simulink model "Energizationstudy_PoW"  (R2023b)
settings: Solver=ode15s  StartTime=0.0  StopTime=25  RelTol=1e-3
PreLoadFcn:
  | Ts=50e-6;
undefined symbols (not defined in the file or in its folder): DiscIntNeverNeededParam, find_system
libraries: spsThreePhaseVIMeasurementLib x11, spsBreakerLib x6, spsabctodq0Lib x6, slpidlib x4, spsFirstOrderFilterLib x3, spsPower3phInstantaneousLib x3, simulink x3, spsThreePhaseBreakerLib x3, spsThreePhaseSeriesRLCBranchLib x2, simulink_extras x2, spsStairGeneratorLib x2, spsThreePhaseSeriesRLCLoadLib x2
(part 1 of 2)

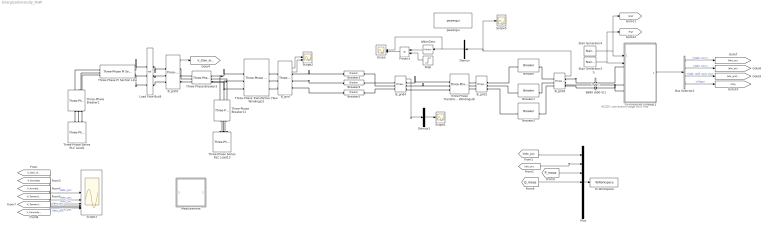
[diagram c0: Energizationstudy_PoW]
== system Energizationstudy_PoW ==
  note: AC/DC conversion stage 80.0 MW
  note: Ts
  B690 (690 V)1 : spsThreePhaseVIMeasurementLib/Three-Phase V-I Measurement  VoltageMeasurement=phase-to-ground  SetLabelV=on  LabelV=Vabc_B575  Vpu=off  VpuLL=off  CurrentMeasurement=yes  SetLabelI=on  LabelI=Iabc_B575  Ipu=off  Pbase=5*2e6/0.9  Vbase=575  OutputType=Complex  PhasorSimulation=off  PSBequivalent=0
  B_grid : spsThreePhaseVIMeasurementLib/Three-Phase V-I Measurement  VoltageMeasurement=phase-to-ground  SetLabelV=off  LabelV=Vabc  Vpu=on  VpuLL=off  CurrentMeasurement=yes  SetLabelI=off  LabelI=Iabc  Ipu=on  Pbase=5e6  Vbase=66e3  OutputType=Complex  PhasorSimulation=off  PSBequivalent=0
  B_grid1 : spsThreePhaseVIMeasurementLib/Three-Phase V-I Measurement  VoltageMeasurement=phase-to-ground  SetLabelV=off  LabelV=Vabc  Vpu=on  VpuLL=off  CurrentMeasurement=yes  SetLabelI=off  LabelI=Iabc  Ipu=on  Pbase=100e6  Vbase=690  OutputType=Complex  PhasorSimulation=off  PSBequivalent=0
  B_grid2 : spsThreePhaseVIMeasurementLib/Three-Phase V-I Measurement  VoltageMeasurement=phase-to-ground  SetLabelV=off  LabelV=Vabc  Vpu=on  VpuLL=off  CurrentMeasurement=no  SetLabelI=off  LabelI=Iabc  Ipu=off  Pbase=5e6  Vbase=132e3  OutputType=Complex  PhasorSimulation=off  PSBequivalent=0
  B_grid3 : spsThreePhaseVIMeasurementLib/Three-Phase V-I Measurement  VoltageMeasurement=phase-to-ground  SetLabelV=off  LabelV=Vabc  Vpu=on  VpuLL=off  CurrentMeasurement=yes  SetLabelI=off  LabelI=Iabc  Ipu=on  Pbase=100e6  Vbase=690  OutputType=Complex  PhasorSimulation=off  PSBequivalent=0
  B_grid4 : spsThreePhaseVIMeasurementLib/Three-Phase V-I Measurement  VoltageMeasurement=phase-to-ground  SetLabelV=off  LabelV=Vabc  Vpu=on  VpuLL=off  CurrentMeasurement=yes  SetLabelI=off  LabelI=Iabc  Ipu=on  Pbase=100e6  Vbase=690  OutputType=Complex  PhasorSimulation=off  PSBequivalent=0
  Breaker : spsBreakerLib/Breaker  InitialState=0  SwitchingTimes=2.0167  External=off  BreakerResistance=0.000001  SnubberResistance=1e6  SnubberCapacitance=1e7  Measurements=None  MoreParameters=on  NoBreakLoop=off
  Breaker1 : spsBreakerLib/Breaker  InitialState=0  SwitchingTimes=2.0117  External=off  BreakerResistance=0.0000001  SnubberResistance=1e6  SnubberCapacitance=1e7  Measurements=None  MoreParameters=on  NoBreakLoop=off
  Breaker2 : spsBreakerLib/Breaker  InitialState=0  SwitchingTimes=2.0117+(0.02/4)  External=off  BreakerResistance=0.0000001  SnubberResistance=1e6  SnubberCapacitance=1e7  Measurements=None  MoreParameters=on  NoBreakLoop=off
  Breaker3 : spsBreakerLib/Breaker  InitialState=0  SwitchingTimes=3.012+0.02/4  External=off  BreakerResistance=0.000001  SnubberResistance=1e6  SnubberCapacitance=1e7  Measurements=None  MoreParameters=on  NoBreakLoop=off
  Breaker4 : spsBreakerLib/Breaker  InitialState=0  SwitchingTimes=3.012  External=off  BreakerResistance=0.000001  SnubberResistance=1e6  SnubberCapacitance=1e7  Measurements=None  MoreParameters=on  NoBreakLoop=off
  Breaker5 : spsBreakerLib/Breaker  InitialState=0  SwitchingTimes=3.012+0.02/4  External=off  BreakerResistance=0.000001  SnubberResistance=1e6  SnubberCapacitance=1e7  Measurements=None  MoreParameters=on  NoBreakLoop=off
  Bus Selector1 : BusSelector  OutputSignals=Vabc_pcc,Iabc_pcc,Iabc_grid_conv_pu,Freq
  Demux : Demux  Outputs=3
  Demux1 : Demux  Outputs=3
  Grid forming inverter1 : Subsystem  LoadFcn=%find_system(gcs,'FollowLinks', 'on', 'LookUnderMasks', 'all');  mask(Grid forming inverter){Vnom=690, fnom=50, Pnom=100e6, Lf=95e-6/20, Rf=10e-3/20, Cf=20*1e-3, Vdc_nom=2000, Innerloops=Inner loops, Kp_cc=0.1425/20, Ki_cc=15/20, Kffv=1, Kp_vc=20*14.25, Ki_vc=20*1500, Kffi=0.9, Virtualimpedance=No virtual impedance, Rvir=0.15, Lvir=50e-5/20, ControlType=Virtual Synchronous Machine, mp=(0.7855e-6)/(2*3.14*50*20), nq=0.5*4.3125e-07/20, Ki_q=1e-4, tau=0.001, Ts=5e-5}
      mask prompts: Vnom "Grid-side converter nominal AC voltage (V):"; fnom "Grid frequency (Hz)"; Pnom "Nominal power (VA)"; Lf "Filter inductance (H)"; Rf "Filter resistance (Ω)"; Cf "Filter capacitor (F):"; Vdc_nom "Nominal DC bus voltage (V)"; Innerloops "Inner loops"; Kp_cc "Proportional gain of the current controller"; Ki_cc "Integral gain of the current controller"; Kffv "Voltage feed-forward"; Kp_vc "Proportional gain of the voltage controller"; Ki_vc "Integral gain of the voltage controller"; Kffi "Current feed-forward"; Virtualimpedance "Virtual impedance"; Rvir "Resistance of the virtual impedance"; Lvir "Inductance of the virtual impedance"; ControlType "Primary control"; mp "P - ω Droop coefficient"; nq "Q - V Droop coefficient"; Ki_q "Integral gain of the reactive power controller"; tau "Filter time constant (s)"; Ts "Sample time (s):"
      mask help: This block implements a model of a grid forming inverter with either droop or virtual synchronous generator control.
      mask init:
      | % Converters data
      | Q_filter=50;
      | 
      | % Controller data
      | Freq_filter=10000;   %Hz
      | Zeta_filter=0.707;
      | Mod_index_max=1.1;
      | T_speed=5;      %Speed reference time constant (s)
      | Iq_ref_limit_time_constant=0.3; %(s)
      | Current_reg_output_limit=1.1;   %(pu)
      | Var_reg_output_hi_limit=1.1;    %(pu)
      | Var_reg_output_low_limit=0.9;   %(pu)
      | Pitch_time_constant=0.01;       %(s)
      | Vf_limit=10;    %Field voltage limit (pu)
      | Freq_sawtooth=2000; %Hz, Boost converter
      | Freq_PWM=3000; %Hz, Inverter
      | Ts_snub=50e-6;  %Sample time to compute snubber resistance
  IsNonZero : simulink/Logic and Bit Operations/Compare To Zero  relop=~=  OutDataTypeStr=boolean
  Load Flow Bus9 : spsLoadFlowBusLib/Load Flow Bus  LConnTagsString=a|b|c  RConnTagsString=a|b|c  Phases=ABC  Connectors=on both sides  ID=Glen Innes 132  Vbase=132e3  Vref=1  Vangle=0  VLF=1  VLFb=1  VLFc=1  angleLF=0  angleLFb=0  angleLFc=0
  Measurement : Subsystem
  Mux : Mux  Inputs=7
  Product : Product
  Scope : Scope  NumInputPorts=2
  Scope1 : Scope
  Scope2 : Scope  NumInputPorts=3
  Scope3 : Scope  NumInputPorts=6
  Scope5 : Scope
  Stair Generator3 : spsStairGeneratorLib/Stair Generator  t=[0]  e=[0]  Ts=0
  Stair Generator4 : spsStairGeneratorLib/Stair Generator  t=[10]  e=[100]  Ts=0
  Step : Step  SampleTime=0
  Three-Phase PI Section Line : spsThreePhasePISectionLineLib/Three-Phase PI Section Line  LConnTagsString=a|b|c  RConnTagsString=A|B|C  Length=1  Frequency=50  Resistances=[14.13/100 44.25/100]  Inductances=[0.0012/100 00.0036/100]  Capacitances=[ 0.0865e-5/100 0.0642e-5/100]
  Three-Phase Series RLC Load1 : spsThreePhaseSeriesRLCLoadLib/Three-Phase Series RLC Load  LConnTagsString=A|B|C  Configuration=Y (grounded)  NominalVoltage=(132000)*1  Vabc=[1e3 1e3 1e3]  Vabcp=[1e3 1e3 1e3]  NominalFrequency=50  UnbalancedPower=off  ActivePower=10e6  InductivePower=0  CapacitivePower=0  Pabc=[10e3 9e3 11e3]  QLabc=[100 90 110]  QCabc=[100 90 110]  Pabcp=[10e3 9e3 11e3]  QLabcp=[100 90 110]  QCabcp=[100 90 110]  Measurements=None  LoadType=constant PQ
  Three-Phase Series RLC Load13 : spsThreePhaseSeriesRLCLoadLib/Three-Phase Series RLC Load  LConnTagsString=A|B|C  Configuration=Y (grounded)  NominalVoltage=(132000)*1  Vabc=[1e3 1e3 1e3]  Vabcp=[1e3 1e3 1e3]  NominalFrequency=50  UnbalancedPower=off  ActivePower=12500  InductivePower=0  CapacitivePower=0  Pabc=[10e3 9e3 11e3]  QLabc=[100 90 110]  QCabc=[100 90 110]  Pabcp=[10e3 9e3 11e3]  QLabcp=[100 90 110]  QCabcp=[100 90 110]  Measurements=None  LoadType=constant PQ
  Three-Phase Transformer (Two Windings)2 : spsThreePhaseTransformerTwoWindingsLib/Three-Phase Transformer (Two Windings)  Winding1Connection=Yg  Winding2Connection=Yg  CoreType=Three-limb core (core-type)  SetSaturation=on  Hysteresis=off  DataFile='hysteresis'  SetInitialFlux=on  Measurements=All measurements (V I Fluxes)  UNITS=pu  NominalPower=[ 100e6 , 50 ]  Winding1=[132e3 , 0.000 , 0.09 ]  Winding2=[ 66e3 , 0.000 , 0.09 ]  Rm=500  Lm=500  L0=0.5  Saturation=[ 0,0 ; 0.0024,1.2 ; 1.0,1.52 ]  InitialFluxes=[-0.7 0 0.7]  BreakLoop=off  DiscreteSolver=Trapezoidal robust  DataType=off  TransfoNumber=1
  Three-Phase Transformer (Two Windings)6 : spsThreePhaseTransformerTwoWindingsLib/Three-Phase Transformer (Two Windings)  Winding1Connection=Yg  Winding2Connection=Yg  CoreType=Three-limb core (core-type)  SetSaturation=on  Hysteresis=off  DataFile='hysteresis'  SetInitialFlux=on  Measurements=All measurements (V I Fluxes)  UNITS=pu  NominalPower=[ 100e6 , 50 ]  Winding1=[66e3 , 0.002 , 0.08 ]  Winding2=[ 690 , 0.002 , 0.08 ]  Rm=500  Lm=500  L0=0.5  Saturation=[ 0,0 ; 0.0024,1.2 ; 1.0,1.52 ]  InitialFluxes=[-0.7 0 0.7]  BreakLoop=off  DiscreteSolver=Trapezoidal robust  DataType=off  TransfoNumber=1
  Three-Phase Breaker1 : spsThreePhaseBreakerLib/Three-Phase Breaker  InitialState=open  SwitchA=on  SwitchB=on  SwitchC=on  SwitchTimes=[120]  External=off  BreakerResistance=1e-10  SnubberResistance=1e10  SnubberCapacitance=inf  Measurements=None
  Three-Phase Breaker11 : spsThreePhaseBreakerLib/Three-Phase Breaker  InitialState=open  SwitchA=on  SwitchB=on  SwitchC=on  SwitchTimes=[120]  External=off  BreakerResistance=1e-10  SnubberResistance=1e10  SnubberCapacitance=inf  Measurements=Breaker currents
  Three-Phase Breaker3 : spsThreePhaseBreakerLib/Three-Phase Breaker  InitialState=open  SwitchA=on  SwitchB=on  SwitchC=on  SwitchTimes=[120]  External=off  BreakerResistance=1e-10  SnubberResistance=1e10  SnubberCapacitance=inf  Measurements=None
  To Workspace : ToWorkspace  VariableName=simout  SaveFormat=Timeseries  SampleTime=-1
  powergui : spspowerguiLib/powergui  SimulationMode=Discrete  SampleTime=5e-5  frequency=50  Iterations=50  frequencyindice=0  Pbase=100e6  ErrMax=1e-4  UnitsV=kV  UnitsW=MW  buscounter=0  FunctionMessages=off  echomessages=off  EnableUseOfTLC=off  CurrentSourceSwitches=off  DisableSnubberDevices=off  DisableRonSwitches=off  DisableVfSwitches=off  DisplayEquations=off  AutomaticDiscreteSolvers=off  SolverType=Tustin  Interpol=off  ExternalGateDelay=off  methode=off  Ts=0  x0status=blocks  SPID=off  SwTol=0  HookPort=off  NonlinearTolerance=1e-4  nMaxIteration=100  ContinueOnMaxIteration=off  RestoreLinks=warning  ResistiveCurrentMeasurement=off  Frange=[0:2:500]  Ylog=off  Xlog=on  ShowGrid=off  save=off  variable=ZData  structure=0  ZoomFFT=on  StartTime=0.0  cycles=1  DisplayStyle=1  fundamental=60  FreqAxis=off  MaxFrequency=1000  frequencyindicesteady=1  RmsSteady=1  display=off
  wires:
  B_grid/1 -> Scope2/1
  B_grid/2 -> Scope2/3
  [Iabc_pcc] -> Mux/2
  Mux/1 -> To Workspace/1
  [Vabc_pcc] -> Mux/1
  B_grid2/1 -> [V_Glen_Innes]
  [V_Glen_Innes] -> Scope3/1  "Vabc_pcc"
  [V_Armidale] -> Scope3/2  "Vabc_pcc"
  [V_Armidale_330] -> Scope3/3  "Vabc_pcc"
  [V_Tamworth_330] -> Scope3/4  "Vabc_pcc"
  [V_Tamworth_132] -> Scope3/5  "Vabc_pcc"
  [V_Gunnedah_132] -> Scope3/6  "Vabc_pcc"
  [Q_meas] -> Mux/4
  [P_meas] -> Mux/3
  Bus Selector1/2 -> [Iabc_pcc]  "<Iabc_pcc>"
  Stair Generator3/1 -> [Pref], Grid forming inverter1/2(Pref_pu)
  Bus Selector1/3 -> [Iabc_grid_conv_pu]  "<Iabc_grid_conv_pu>"
  Grid forming inverter1/1(m) -> Bus Selector1/1
  Bus Selector1/4 -> [Freq]  "<Freq>"
  Bus Selector1/1 -> [Vabc_pcc]  "<Vabc_pcc>"
  Stair Generator4/1 -> [Qref], Grid forming inverter1/1(Qref_pu)
  Demux/2 -> IsNonZero/1, Scope/1
  IsNonZero/1 -> Product/1
  Step/1 -> Product/2
  Product/1 -> Scope/2
  B_grid3/1 -> Scope5/1, Demux/1
  Demux1/2 -> Scope1/1
  B_grid4/1 -> Demux1/1
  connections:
  B_grid/LConn1 -- Three-Phase Transformer (Two Windings)2/RConn1
  B_grid/LConn2 -- Three-Phase Transformer (Two Windings)2/RConn2
  B_grid/LConn3 -- Three-Phase Transformer (Two Windings)2/RConn3
  Three-Phase Breaker3/RConn1 -- Three-Phase Breaker11/LConn1 -- Three-Phase Transformer (Two Windings)2/LConn1
  Three-Phase Breaker11/RConn3 -- Three-Phase Series RLC Load13/LConn1
  Three-Phase Breaker11/RConn2 -- Three-Phase Series RLC Load13/LConn2
  Three-Phase Breaker11/RConn1 -- Three-Phase Series RLC Load13/LConn3
  Three-Phase PI Section Line/LConn2 -- Three-Phase Breaker1/LConn2
  Three-Phase Breaker1/LConn1 -- Three-Phase PI Section Line/LConn1
  Three-Phase Breaker1/LConn3 -- Three-Phase PI Section Line/LConn3
  Three-Phase PI Section Line/RConn1 -- Load Flow Bus9/RConn1
  Three-Phase PI Section Line/RConn2 -- Load Flow Bus9/RConn2
  Three-Phase PI Section Line/RConn3 -- Load Flow Bus9/RConn3
  Three-Phase Transformer (Two Windings)6/RConn1 -- B_grid1/LConn1
  Three-Phase Transformer (Two Windings)6/RConn2 -- B_grid1/LConn2
  Three-Phase Transformer (Two Windings)6/RConn3 -- B_grid1/LConn3
  Load Flow Bus9/LConn1 -- B_grid2/LConn1
  Load Flow Bus9/LConn2 -- B_grid2/LConn2
  Load Flow Bus9/LConn3 -- B_grid2/LConn3
  B_grid2/RConn1 -- Three-Phase Breaker3/LConn1
  B_grid2/RConn2 -- Three-Phase Breaker3/LConn2
  B_grid2/RConn3 -- Three-Phase Breaker3/LConn3
  Three-Phase Transformer (Two Windings)2/LConn2 -- Three-Phase Breaker11/LConn2 -- Three-Phase Breaker3/RConn2
  Three-Phase Breaker3/RConn3 -- Three-Phase Breaker11/LConn3 -- Three-Phase Transformer (Two Windings)2/LConn3
  Three-Phase Series RLC Load1/LConn3 -- Three-Phase Breaker1/RConn1
  Three-Phase Series RLC Load1/LConn2 -- Three-Phase Breaker1/RConn2
  Three-Phase Series RLC Load1/LConn1 -- Three-Phase Breaker1/RConn3
  B_grid1/RConn1 -- Breaker/LConn1
  Breaker1/LConn1 -- B_grid1/RConn2
  Breaker2/LConn1 -- B_grid1/RConn3
  B_grid/RConn1 -- Breaker3/LConn1
  B_grid/RConn2 -- Breaker4/LConn1
  B_grid/RConn3 -- Breaker5/LConn1
  Grid forming inverter1/LConn2 -- B690 (690 V)1/RConn2
  Grid forming inverter1/LConn1 -- B690 (690 V)1/RConn1
  Grid forming inverter1/LConn3 -- B690 (690 V)1/RConn3
  B_grid3/RConn1 -- B690 (690 V)1/LConn1
  B_grid3/RConn2 -- B690 (690 V)1/LConn2
  B_grid3/RConn3 -- B690 (690 V)1/LConn3
  B_grid4/RConn1 -- Three-Phase Transformer (Two Windings)6/LConn1
  B_grid4/RConn2 -- Three-Phase Transformer (Two Windings)6/LConn2
  B_grid4/RConn3 -- Three-Phase Transformer (Two Windings)6/LConn3
  Breaker3/RConn1 -- B_grid4/LConn1
  Breaker4/RConn1 -- B_grid4/LConn2
  Breaker5/RConn1 -- B_grid4/LConn3
  Breaker/RConn1 -- B_grid3/LConn1
  Breaker1/RConn1 -- B_grid3/LConn2
  Breaker2/RConn1 -- B_grid3/LConn3

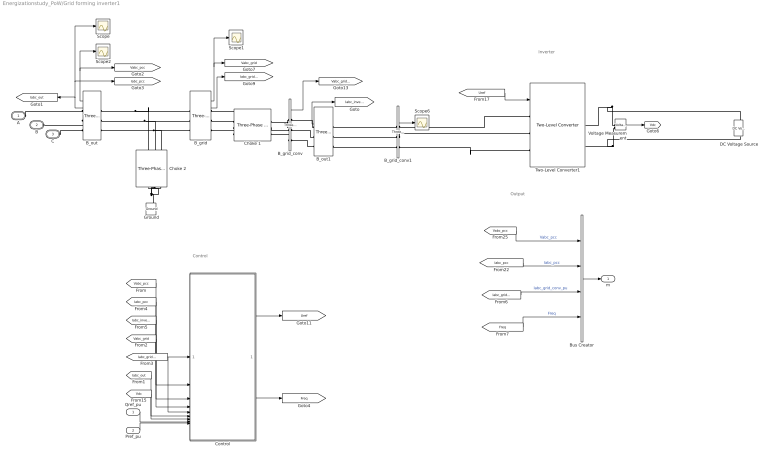
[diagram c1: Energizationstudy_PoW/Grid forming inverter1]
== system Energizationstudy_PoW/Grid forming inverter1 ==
  note: Control
  note: Inverter
  note: Output
  Qref_pu : Inport
  Pref_pu : Inport  Port=2
  B_grid : spsThreePhaseVIMeasurementLib/Three-Phase V-I Measurement  VoltageMeasurement=phase-to-ground  SetLabelV=off  LabelV=Vabc  Vpu=on  VpuLL=off  CurrentMeasurement=yes  SetLabelI=off  LabelI=Iabc  Ipu=on  Pbase=5e6  Vbase=690  OutputType=Complex  PhasorSimulation=off  PSBequivalent=0
  B_grid_conv : spsThreePhaseVIMeasurementLib/Three-Phase V-I Measurement  VoltageMeasurement=phase-to-ground  SetLabelV=off  LabelV=Vabc  Vpu=on  VpuLL=off  CurrentMeasurement=yes  SetLabelI=off  LabelI=Iabc  Ipu=off  Pbase=Pnom  Vbase=Vnom  OutputType=Complex  PhasorSimulation=off  PSBequivalent=0
  B_grid_conv1 : spsThreePhaseVIMeasurementLib/Three-Phase V-I Measurement  VoltageMeasurement=phase-to-ground  SetLabelV=off  LabelV=Vabc  Vpu=off  VpuLL=off  CurrentMeasurement=yes  SetLabelI=off  LabelI=Iabc  Ipu=off  Pbase=Pnom  Vbase=Vnom  OutputType=Complex  PhasorSimulation=off  PSBequivalent=0
  B_out : spsThreePhaseVIMeasurementLib/Three-Phase V-I Measurement  VoltageMeasurement=phase-to-ground  SetLabelV=off  LabelV=Vabc  Vpu=off  VpuLL=off  CurrentMeasurement=yes  SetLabelI=off  LabelI=Iabc  Ipu=off  Pbase=5e6  Vbase=690  OutputType=Complex  PhasorSimulation=off  PSBequivalent=0
  B_out1 : spsThreePhaseVIMeasurementLib/Three-Phase V-I Measurement  VoltageMeasurement=phase-to-ground  SetLabelV=off  LabelV=Vabc  Vpu=off  VpuLL=off  CurrentMeasurement=yes  SetLabelI=off  LabelI=Iabc  Ipu=off  Pbase=5e6  Vbase=690  OutputType=Complex  PhasorSimulation=off  PSBequivalent=0
  Bus Creator : BusCreator  Inputs=4
  Choke 1 : spsThreePhaseSeriesRLCBranchLib/Three-Phase Series RLC Branch  LConnTagsString=A|B|C  RConnTagsString=A|B|C  BranchType=RL  Resistance=Rf  Inductance=Lf  Capacitance=[]  Measurements=None
  Choke 2 : spsThreePhaseSeriesRLCBranchLib/Three-Phase Series RLC Branch  LConnTagsString=A|B|C  RConnTagsString=A|B|C  BranchType=C  Resistance=10e-3  Inductance=95e-6  Capacitance=Cf  Measurements=None
  Control : Subsystem
  DC Voltage Source : spsDCVoltageSourceLib/DC Voltage Source  Amplitude=Vdc_nom  Measurements=None
  Ground : spsGroundLib/Ground  LConnTagsString=a
  Scope{,1..2,6} (4 alike) : Scope
  Two-Level Converter1 : spsTwoLevelConverterLib/Two-Level Converter  ModelType=Average model (No rectifier mode)  Ron=1e-3  Rs=1e6  Cs=inf  Vforward=[0,0]  Ron_Diode=1e-3  Rs_Diode=1e6  Cs_Diode=inf  Vf_Diode=1e-3  Rs_CurrentSource=inf  Ron_ACsource=1e-3
  Voltage Measurement : spsVoltageMeasurementLib/Voltage Measurement  PhasorSimulation=off  OutputType=Complex  PSBequivalent=0
  A : PMIOPort  Tag=PMCPort  Side=Left
  B : PMIOPort  Tag=PMCPort  Port=2  Side=Left
  C : PMIOPort  Tag=PMCPort  Port=3  Side=Left
  m : Outport  VectorParamsAs1DForOutWhenUnconnected=off
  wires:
  B_grid_conv/1 -> [Vabc_grid_conv]
  B_grid/1 -> Scope1/1, [Vabc_grid]
  B_grid/2 -> [Iabc_grid_conv]
  [Vabc_grid] -> Control/4(Vabc_grid)
  [Iabc_grid_conv] -> Control/5(Iabc_grid_conv)
  [Vdc] -> Control/7(Vdc)
  Qref_pu/1 -> Control/8(Qref)
  Control/1(Uref) -> [Uref]
  [Uref] -> Two-Level Converter1/1
  [Vabc_pcc] -> Bus Creator/1  "Vabc_pcc"
  Bus Creator/1 -> m/1
  [Iabc_pcc] -> Bus Creator/2  "Iabc_pcc"
  [Iabc_grid_conv] -> Bus Creator/3  "Iabc_grid_conv_pu"
  [Iabc_out] -> Control/6(Iabc_out)
  Pref_pu/1 -> Control/9(Pref_pu)
  Voltage Measurement/1 -> [Vdc]
  B_out/1 -> [Vabc_pcc], Scope2/1
  [Vabc_pcc] -> Control/1(Vabc_pcc)
  [Iabc_pcc] -> Control/2(Iabc_pcc)
  [Iabc_inverter] -> Control/3(Iabc_inverter)
  B_out1/2 -> [Iabc_inverter]
  B_grid_conv1/2 -> Scope6/1
  B_out/2 -> Scope/1, [Iabc_pcc], [Iabc_out]
  Control/2(Freq) -> [Freq]
  [Freq] -> Bus Creator/4  "Freq"
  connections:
  B_out/LConn1 -- Choke 2/LConn1 -- B_grid/LConn1
  B_out/LConn2 -- Choke 2/LConn2 -- B_grid/LConn2
  B_out/LConn3 -- Choke 2/LConn3 -- B_grid/LConn3
  Voltage Measurement/LConn2 -- DC Voltage Source/LConn1 -- Two-Level Converter1/RConn2
  Voltage Measurement/LConn1 -- DC Voltage Source/RConn1 -- Two-Level Converter1/RConn1
  C/RConn1 -- B_out/RConn3
  B_out/RConn2 -- B/RConn1
  A/RConn1 -- B_out/RConn1
  Two-Level Converter1/LConn1 -- B_grid_conv1/RConn1
  B_grid_conv1/RConn2 -- Two-Level Converter1/LConn2
  B_grid_conv1/RConn3 -- Two-Level Converter1/LConn3
  B_out1/LConn1 -- B_grid_conv1/LConn1
  B_out1/LConn3 -- B_grid_conv1/LConn3
  Choke 2/RConn2 -- Ground/LConn1 -- Choke 2/RConn1 -- Choke 2/RConn3
  B_grid_conv1/LConn2 -- B_out1/LConn2
  B_out1/RConn1 -- B_grid_conv/RConn1
  B_out1/RConn2 -- B_grid_conv/RConn2
  B_out1/RConn3 -- B_grid_conv/RConn3
  Choke 1/RConn2 -- B_grid_conv/LConn2
  B_grid_conv/LConn1 -- Choke 1/RConn1
  B_grid_conv/LConn3 -- Choke 1/RConn3
  Choke 1/LConn1 -- B_grid/RConn1
  Choke 1/LConn2 -- B_grid/RConn2
  Choke 1/LConn3 -- B_grid/RConn3

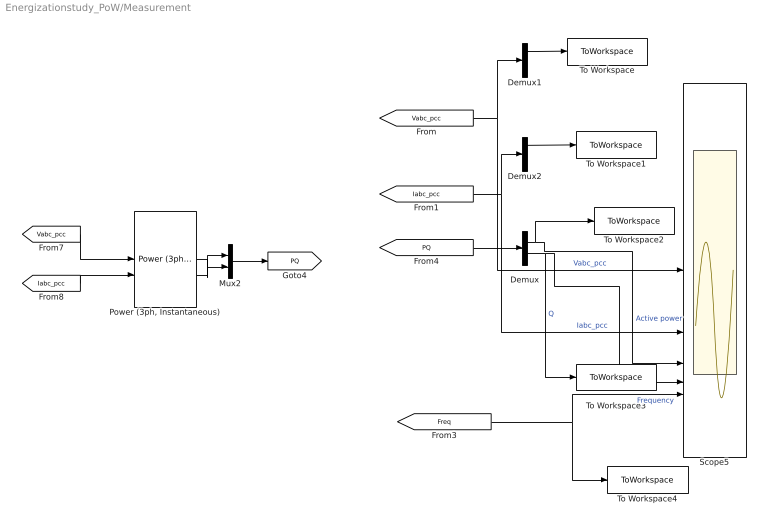
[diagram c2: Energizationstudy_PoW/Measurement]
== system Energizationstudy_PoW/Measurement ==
  Demux : Demux  Outputs=2
  Demux1 : Demux  Outputs=3
  Demux2 : Demux  Outputs=3
  Mux2 : Mux  Inputs=2
  "Power (3ph, Instantaneous)" : spsPower3phInstantaneousLib/Power (3ph, Instantaneous)
  Scope5 : Scope  NumInputPorts=5
  To Workspace : ToWorkspace  VariableName=Va  SaveFormat=Timeseries  SampleTime=-1
  To Workspace1 : ToWorkspace  VariableName=Ia  SaveFormat=Timeseries  SampleTime=-1
  To Workspace2 : ToWorkspace  VariableName=P  SaveFormat=Timeseries  SampleTime=-1
  To Workspace3 : ToWorkspace  VariableName=Q  SaveFormat=Timeseries  SampleTime=-1
  To Workspace4 : ToWorkspace  VariableName=F  SaveFormat=Timeseries  SampleTime=-1
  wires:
  [PQ] -> Demux/1
  Demux/2 -> To Workspace3/1, Scope5/4  "Q"
  Demux/1 -> To Workspace2/1, Scope5/3  "Active power"
  "Power (3ph, Instantaneous)"/2 -> Mux2/2
  [Vabc_pcc] -> "Power (3ph, Instantaneous)"/1
  [Iabc_pcc] -> "Power (3ph, Instantaneous)"/2
  "Power (3ph, Instantaneous)"/1 -> Mux2/1
  Mux2/1 -> [PQ]
  [Freq] -> To Workspace4/1, Scope5/5  "Frequency"
  [Vabc_pcc] -> Demux1/1, Scope5/1  "Vabc_pcc"
  [Iabc_pcc] -> Demux2/1, Scope5/2  "Iabc_pcc"
  Demux1/1 -> To Workspace/1
  Demux2/1 -> To Workspace1/1

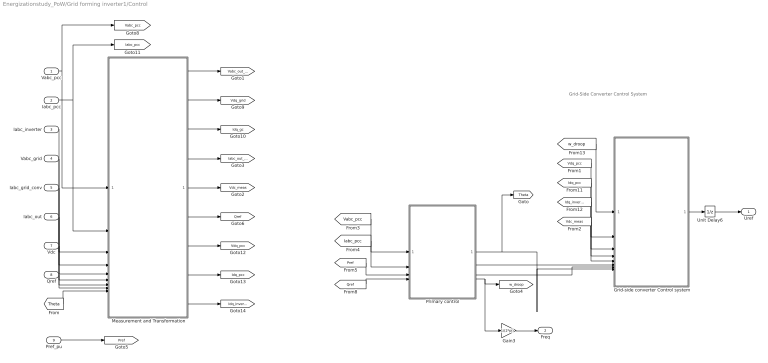
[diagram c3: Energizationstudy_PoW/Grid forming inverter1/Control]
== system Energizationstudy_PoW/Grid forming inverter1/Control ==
  note: Grid-Side Converter Control System
  Vabc_pcc : Inport
  Iabc_pcc : Inport  Port=2
  Iabc_inverter : Inport  Port=3
  Vabc_grid : Inport  Port=4
  Iabc_grid_conv : Inport  Port=5
  Iabc_out : Inport  Port=6
  Vdc : Inport  Port=7
  Qref : Inport  Port=8
  Pref_pu : Inport  Port=9
  Gain3 : Gain  Gain=1/(2*pi)
  Grid-side converter Control system : Subsystem
  Measurement and Transformation : Subsystem
  Primary control : Subsystem  Variant=on  VariantControl=Choice
  Unit Delay6 : UnitDelay  SampleTime=Ts  HasFrameUpgradeWarning=on
  Uref : Outport  VectorParamsAs1DForOutWhenUnconnected=off
  Freq : Outport  Port=2  VectorParamsAs1DForOutWhenUnconnected=off
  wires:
  [Vdq_pcc] -> Grid-side converter Control system/2(Vdq_pcc)
  [Vdc_meas] -> Grid-side converter Control system/5(Vdc)
  Grid-side converter Control system/1(Uctrl_inverter) -> Unit Delay6/1
  Unit Delay6/1 -> Uref/1
  Vabc_grid/1 -> Measurement and Transformation/4(Vabc_grid)
  Iabc_grid_conv/1 -> Measurement and Transformation/5(Iabc_gc)
  Vdc/1 -> Measurement and Transformation/7(Vdc)
  Qref/1 -> Measurement and Transformation/8(Qref)
  Measurement and Transformation/2(Vdq_grid) -> [Vdq_grid]
  Measurement and Transformation/3(Idq_gc) -> [Idq_gc]
  Measurement and Transformation/5(Vdc_meas) -> [Vdc_meas]
  Measurement and Transformation/6("Qref ") -> [Qref]
  Iabc_out/1 -> Measurement and Transformation/6(Iabc_out)
  [Theta] -> Measurement and Transformation/9(Theta)
  Measurement and Transformation/4(I_abc_out) -> [Iabc_out_pu]
  Measurement and Transformation/1(V_abc_grid) -> [Vabc_out_pu]
  Pref_pu/1 -> [Pref]
  Vabc_pcc/1 -> [Vabc_pcc], Measurement and Transformation/1(Vabc_pcc)
  Iabc_pcc/1 -> [Iabc_pcc], Measurement and Transformation/2(Iabc_pcc)
  Iabc_inverter/1 -> Measurement and Transformation/3(Iabc_inverter)
  [Idq_pcc] -> Grid-side converter Control system/3(Idq_pcc)
  [Idq_inverter] -> Grid-side converter Control system/4(Idq_inverter)
  Measurement and Transformation/7(Vdq_pcc) -> [Vdq_pcc]
  Measurement and Transformation/8(Idq_pcc) -> [Idq_pcc]
  Measurement and Transformation/9(Idq_inverter) -> [Idq_inverter]
  [w_droop] -> Grid-side converter Control system/1(w)
  [Vabc_pcc] -> Primary control/1(Vabc_pu)
  [Iabc_pcc] -> Primary control/2(Iabc_pu)
  [Pref] -> Primary control/3(Pref_pu)
  [Qref] -> Primary control/4(Qref_pu)
  Primary control/1(Theta) -> Grid-side converter Control system/8(Theta_PLL), [Theta]
  Primary control/2(Vd_ref) -> Grid-side converter Control system/6(Vd_ref)
  Primary control/3(Vq_ref) -> Grid-side converter Control system/7(Vq_ref)
  Primary control/4(w_droop) -> Gain3/1, [w_droop]
  Gain3/1 -> Freq/1

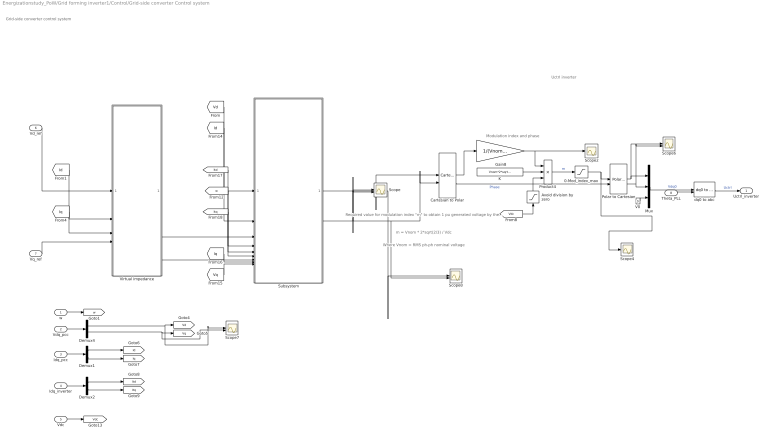
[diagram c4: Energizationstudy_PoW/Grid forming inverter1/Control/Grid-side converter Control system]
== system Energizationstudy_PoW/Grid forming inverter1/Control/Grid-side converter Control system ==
  note: Modulation index and phase
  note: Where Vnom = RMS ph-ph nominal voltage
  note: m = Vnom * 2*sqrt(2/3) / Vdc
  note: Required value for modulation index "m" to obtain 1 pu generated voltage by the converter:
  note: Grid-side converter control system
  note: Uctrl inverter
  w : Inport
  Vdq_pcc : Inport  Port=2
  Idq_pcc : Inport  Port=3
  Idq_inverter : Inport  Port=4
  Vdc : Inport  Port=5
  Vd_ref : Inport  Port=6
  Vq_ref : Inport  Port=7
  Theta_PLL : Inport  Port=8
  0-Mod_index_max : Saturate  UpperLimit=Mod_index_max*0+1.4  LowerLimit=0
  Avoid division by zero : Saturate  UpperLimit=1e6  LowerLimit=1e-6
  Cartesian to Polar : simulink_extras/Transformations/Cartesian to Polar
  Demux1 : Demux  Outputs=2
  Demux2 : Demux  Outputs=2
  Demux4 : Demux  Outputs=2
  Gain8 : Gain  Gain=1/(Vnom*sqrt(2/3))
  K : Constant  Value=Vnom*2*sqrt(2/3)
  Mux : Mux  Inputs=3
  Polar to Cartesian : simulink_extras/Transformations/Polar to Cartesian
  Product4 : Product  Inputs=**/  InputSameDT=on  SaturateOnIntegerOverflow=on
  Scope{,6..8} (4 alike) : Scope  NumInputPorts=2
  Scope2 : Scope
  Scope4 : Scope
  Subsystem : Subsystem  Variant=on  VariantControl=Choice
  V0 : Constant  Value=0
  Virtual impedance : Subsystem  Variant=on  VariantControl=Choice
  dq0 to abc : spsdq0toabcLib/dq0 to abc  Alignment=90 degrees behind phase A axis
  Uctrl_inverter : Outport  VectorParamsAs1DForOutWhenUnconnected=off
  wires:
  0-Mod_index_max/1 -> Polar to Cartesian/1, Scope4/1
  Cartesian to Polar/2 -> Polar to Cartesian/2  "Phase"
  [Vdc] -> Avoid division by zero/1
  Cartesian to Polar/1 -> Gain8/1
  Avoid division by zero/1 -> Product4/3
  K/1 -> Product4/2
  Product4/1 -> 0-Mod_index_max/1  "m"
  Demux4/2 -> Scope7/2, [Vq]
  Demux4/1 -> Scope7/1, [Vd]
  w/1 -> [w]
  Vdq_pcc/1 -> Demux4/1
  Vdc/1 -> [Vdc]
  Idq_pcc/1 -> Demux1/1
  Demux1/1 -> [Id]
  Demux1/2 -> [Iq]
  Demux2/2 -> [Itq]
  Demux2/1 -> [Itd]
  Idq_inverter/1 -> Demux2/1
  Polar to Cartesian/1 -> Mux/1, Scope6/1
  Theta_PLL/1 -> dq0 to abc/2
  V0/1 -> Mux/3
  Polar to Cartesian/2 -> Mux/2, Scope6/2
  Mux/1 -> dq0 to abc/1  "Vdq0"
  dq0 to abc/1 -> Uctrl_inverter/1  "Uctrl"
  Gain8/1 -> Product4/1, Scope2/1
  Vd_ref/1 -> Virtual impedance/1(Vd_ref)
  [Id] -> Virtual impedance/2(Id)
  [Iq] -> Virtual impedance/3(Iq)
  Vq_ref/1 -> Virtual impedance/4(Vq_ref)
  Subsystem/1(Vd inverter) -> Scope/1, Scope8/1, Cartesian to Polar/1
  Subsystem/2(Vq inverter) -> Scope/2, Cartesian to Polar/2, Scope8/2
  [Vd] -> Subsystem/1(Vd)
  [Id] -> Subsystem/2(Id)
  [Vq] -> Subsystem/9(Vq)
  Virtual impedance/1(Vd_ref*) -> Subsystem/3(Vd_ref)
  [Iq] -> Subsystem/8(Iq)
  [Itd] -> Subsystem/4(Itd)
  Virtual impedance/2(Vq_ref*) -> Subsystem/7(Vq_ref)
  [w] -> Subsystem/5(w)
  [Itq] -> Subsystem/6(Itq)

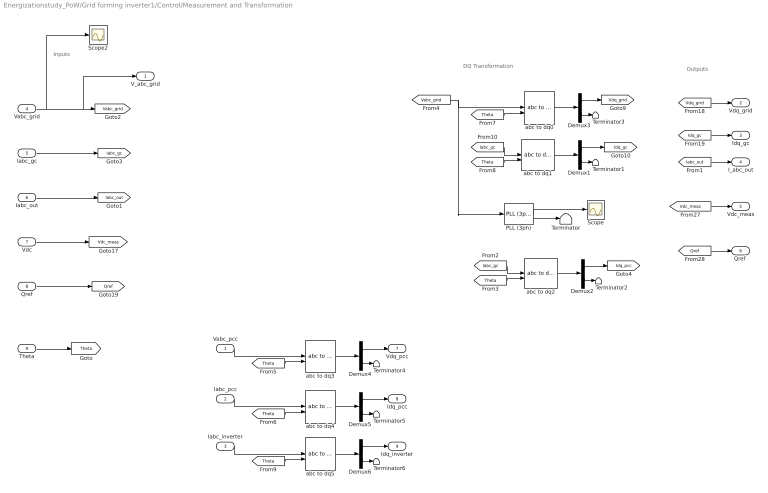
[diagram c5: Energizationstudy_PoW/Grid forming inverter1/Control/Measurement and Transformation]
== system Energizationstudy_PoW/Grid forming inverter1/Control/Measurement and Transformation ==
  note: Inputs
  note: DQ Transformation
  note: Outputs
  Vabc_pcc : Inport
  Iabc_pcc : Inport  Port=2
  Iabc_inverter : Inport  Port=3
  Vabc_grid : Inport  Port=4
  Iabc_gc : Inport  Port=5
  Iabc_out : Inport  Port=6
  Vdc : Inport  Port=7
  Qref : Inport  Port=8
  Theta : Inport  Port=9
  Demux{1..6} (6 alike) : Demux  Outputs=[2 1]
  PLL (3ph) : spsPLL3phLib/PLL (3ph)  Fmin=35  Par_Init=[0, 50]  ParK=[180, 3200, 0]  TcD=1e-4  MaxRateChangeFreq=12  FilterCutOffFreq=25  Ts=Ts  AGC=on
  Scope : Scope
  Scope2 : Scope
  Terminator{,1..6} (7 alike) : Terminator
  abc to dq{0..5} (6 alike) : spsabctodq0Lib/abc to dq0  Alignment=90 degrees behind phase A axis
  V_abc_grid : Outport  VectorParamsAs1DForOutWhenUnconnected=off
  Vdq_grid : Outport  Port=2  VectorParamsAs1DForOutWhenUnconnected=off
  Idq_gc : Outport  Port=3  VectorParamsAs1DForOutWhenUnconnected=off
  I_abc_out : Outport  Port=4  VectorParamsAs1DForOutWhenUnconnected=off
  Vdc_meas : Outport  Port=5  VectorParamsAs1DForOutWhenUnconnected=off
  "Qref " : Outport  Port=6  VectorParamsAs1DForOutWhenUnconnected=off
  Vdq_pcc : Outport  Port=7  VectorParamsAs1DForOutWhenUnconnected=off
  Idq_pcc : Outport  Port=8  VectorParamsAs1DForOutWhenUnconnected=off
  Idq_inverter : Outport  Port=9  VectorParamsAs1DForOutWhenUnconnected=off
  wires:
  Qref/1 -> [Qref]
  Vdc/1 -> [Vdc_meas]
  Iabc_gc/1 -> [Iabc_gc]
  Vabc_grid/1 -> V_abc_grid/1, [Vabc_grid], Scope2/1
  [Qref] -> "Qref "/1
  [Vdc_meas] -> Vdc_meas/1
  [Idq_gc] -> Idq_gc/1
  [Vdq_grid] -> Vdq_grid/1
  Demux1/1 -> [Idq_gc]
  [Iabc_gc] -> abc to dq1/1
  [Theta] -> abc to dq1/2
  [Vabc_grid] -> PLL (3ph)/1, abc to dq0/1
  abc to dq0/1 -> Demux3/1
  abc to dq1/1 -> Demux1/1
  Demux3/2 -> Terminator3/1
  Demux3/1 -> [Vdq_grid]
  Demux1/2 -> Terminator1/1
  Theta/1 -> [Theta]
  Iabc_out/1 -> [Iabc_out]
  [Iabc_out] -> I_abc_out/1
  PLL (3ph)/2 -> Terminator/1
  PLL (3ph)/1 -> Scope/1
  [Theta] -> abc to dq0/2
  Demux2/1 -> [Idq_pcc]
  abc to dq2/1 -> Demux2/1
  [Theta] -> abc to dq2/2
  Demux2/2 -> Terminator2/1
  [Iabc_gc] -> abc to dq2/1
  abc to dq3/1 -> Demux4/1
  [Theta] -> abc to dq3/2
  Demux4/2 -> Terminator4/1
  Demux4/1 -> Vdq_pcc/1
  [Theta] -> abc to dq4/2
  Demux5/2 -> Terminator5/1
  Demux5/1 -> Idq_pcc/1
  abc to dq4/1 -> Demux5/1
  Demux6/2 -> Terminator6/1
  abc to dq5/1 -> Demux6/1
  Demux6/1 -> Idq_inverter/1
  [Theta] -> abc to dq5/2
  Vabc_pcc/1 -> abc to dq3/1
  Iabc_pcc/1 -> abc to dq4/1
  Iabc_inverter/1 -> abc to dq5/1

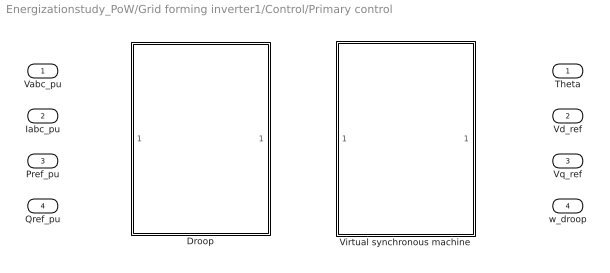
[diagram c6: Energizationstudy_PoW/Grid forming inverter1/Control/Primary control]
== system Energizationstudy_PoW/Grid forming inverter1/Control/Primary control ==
  Vabc_pu : Inport
  Iabc_pu : Inport  Port=2
  Pref_pu : Inport  Port=3
  Qref_pu : Inport  Port=4
  Droop : Subsystem  VariantControl=ControlType == 1
  Virtual synchronous machine : Subsystem  VariantControl=ControlType == 2
  Theta : Outport
  Vd_ref : Outport  Port=2
  Vq_ref : Outport  Port=3
  w_droop : Outport  Port=4

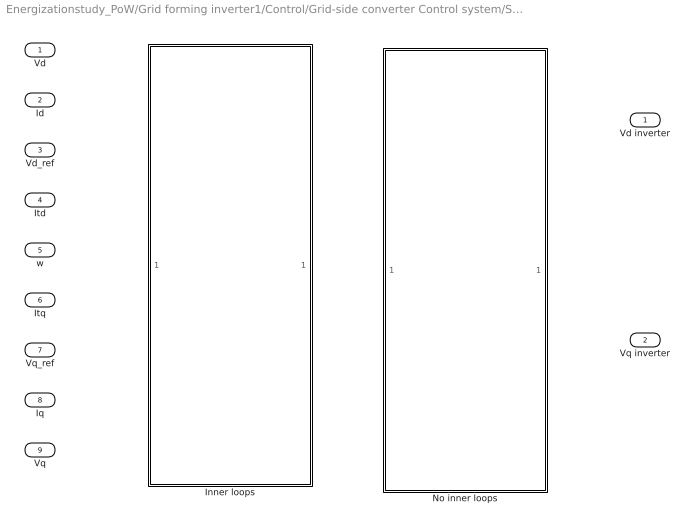
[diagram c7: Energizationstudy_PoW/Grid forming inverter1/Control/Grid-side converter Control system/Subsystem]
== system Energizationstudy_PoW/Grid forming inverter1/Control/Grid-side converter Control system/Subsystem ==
  Vd : Inport
  Id : Inport  Port=2
  Vd_ref : Inport  Port=3
  Itd : Inport  Port=4
  w : Inport  Port=5
  Itq : Inport  Port=6
  Vq_ref : Inport  Port=7
  Iq : Inport  Port=8
  Vq : Inport  Port=9
  Inner loops : Subsystem  VariantControl=Innerloops == 1
  No inner loops : Subsystem  VariantControl=Innerloops == 2
  Vd inverter : Outport
  Vq inverter : Outport  Port=2

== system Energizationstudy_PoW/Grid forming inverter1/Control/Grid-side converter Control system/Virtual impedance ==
  Vd_ref : Inport
  Id : Inport  Port=2
  Iq : Inport  Port=3
  Vq_ref : Inport  Port=4
  No virtual impedance : Subsystem  VariantControl=Virtualimpedance == 2
  Virtual impedance : Subsystem  VariantControl=Virtualimpedance == 1
  Vd_ref* : Outport
  Vq_ref* : Outport  Port=2

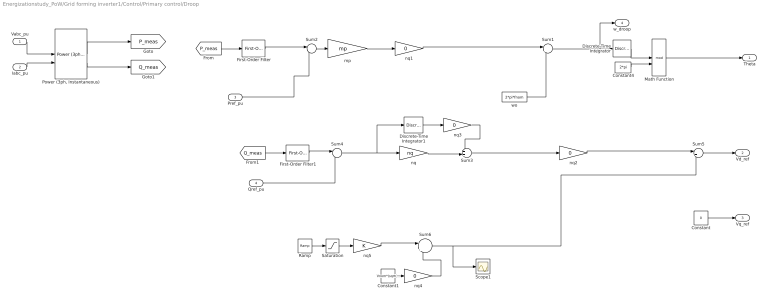
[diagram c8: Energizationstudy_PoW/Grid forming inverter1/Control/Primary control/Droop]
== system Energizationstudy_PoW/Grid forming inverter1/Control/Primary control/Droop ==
  Vabc_pu : Inport
  Iabc_pu : Inport  Port=2
  Pref_pu : Inport  Port=3
  Qref_pu : Inport  Port=4
  Constant : Constant  Value=0
  Constant1 : Constant  Value=Vnom*(sqrt(2/3))
  Constant4 : Constant  Value=2*pi
  Discrete-Time Integrator : DiscreteIntegrator  gainval=1  SampleTime=Ts  ICPrevOutput=DiscIntNeverNeededParam  ICPrevScaledInput=DiscIntNeverNeededParam
  Discrete-Time Integrator1 : DiscreteIntegrator  gainval=Ki_q  SampleTime=Ts  ICPrevOutput=DiscIntNeverNeededParam  ICPrevScaledInput=DiscIntNeverNeededParam
  First-Order Filter : spsFirstOrderFilterLib/First-Order Filter  FilterType=Lowpass  Tc=tau  Ts=Ts  Initialize=off  Vac_Init=[0, 0, 60]  Vdc_Init=0  PlotResponse=off  FreqRange="[0,  200,  1]"
  First-Order Filter1 : spsFirstOrderFilterLib/First-Order Filter  FilterType=Lowpass  Tc=0.0001  Ts=Ts  Initialize=off  Vac_Init=[0, 0, 60]  Vdc_Init=0  PlotResponse=off  FreqRange="[0,  200,  1]"
  Math Function : Math  Operator=mod  SignedPower=on
  "Power (3ph, Instantaneous)" : spsPower3phInstantaneousLib/Power (3ph, Instantaneous)
  Ramp : simulink/Sources/Ramp  slope=563.8/20  start=0  InitialOutput=0
  Saturation : Saturate  UpperLimit=563.5  LowerLimit=0
  Scope1 : Scope
  Sum1 : Sum  Inputs=|++  InputSameDT=on  SaturateOnIntegerOverflow=on
  Sum2 : Sum  Inputs=|-+  InputSameDT=on  SaturateOnIntegerOverflow=on
  Sum3 : Sum  Inputs=++|  InputSameDT=on  SaturateOnIntegerOverflow=on
  Sum4 : Sum  Inputs=|-+  InputSameDT=on  SaturateOnIntegerOverflow=on
  Sum5 : Sum  Inputs=|++  InputSameDT=on  SaturateOnIntegerOverflow=on
  Sum6 : Sum  Inputs=|++
  mp : Gain  Gain=mp
  nq : Gain  Gain=nq
  nq{1..4} (4 alike) : Gain  Gain=0
  nq5 : Gain
  wo : Constant  Value=2*pi*fnom
  Theta : Outport
  Vd_ref : Outport  Port=2
  Vq_ref : Outport  Port=3
  w_droop : Outport  Port=4
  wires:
  Constant4/1 -> Math Function/2
  Discrete-Time Integrator/1 -> Math Function/1
  wo/1 -> Sum1/2
  Sum2/1 -> mp/1
  First-Order Filter/1 -> Sum2/1
  Pref_pu/1 -> Sum2/2
  Vabc_pu/1 -> "Power (3ph, Instantaneous)"/1
  Iabc_pu/1 -> "Power (3ph, Instantaneous)"/2
  "Power (3ph, Instantaneous)"/1 -> [P_meas]
  "Power (3ph, Instantaneous)"/2 -> [Q_meas]
  [P_meas] -> First-Order Filter/1
  Constant/1 -> Vq_ref/1
  Sum6/1 -> Sum5/2, Scope1/1
  nq/1 -> Sum3/2
  Sum4/1 -> Discrete-Time Integrator1/1, nq/1
  [Q_meas] -> First-Order Filter1/1
  First-Order Filter1/1 -> Sum4/1
  Qref_pu/1 -> Sum4/2
  Sum1/1 -> w_droop/1, Discrete-Time Integrator/1
  Math Function/1 -> Theta/1
  Sum5/1 -> Vd_ref/1
  mp/1 -> nq1/1
  nq1/1 -> Sum1/1
  Sum3/1 -> nq2/1
  nq2/1 -> Sum5/1
  Discrete-Time Integrator1/1 -> nq3/1
  nq3/1 -> Sum3/1
  Ramp/1 -> Saturation/1
  Constant1/1 -> nq4/1
  Saturation/1 -> nq5/1
  nq5/1 -> Sum6/1
  nq4/1 -> Sum6/2

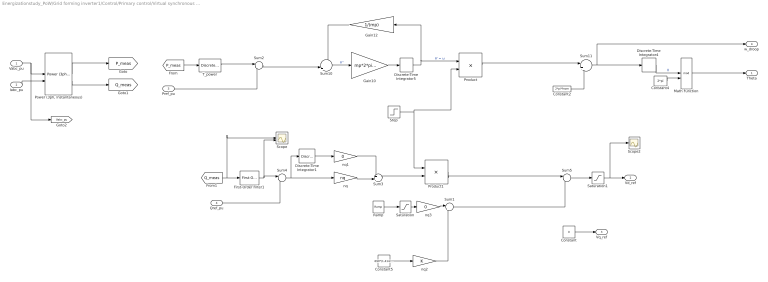
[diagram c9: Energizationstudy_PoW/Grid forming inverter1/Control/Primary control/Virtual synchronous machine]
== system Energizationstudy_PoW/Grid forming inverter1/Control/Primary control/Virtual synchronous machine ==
  Vabc_pu : Inport
  Iabc_pu : Inport  Port=2
  Pref_pu : Inport  Port=3
  Qref_pu : Inport  Port=4
  Constant : Constant  Value=0
  Constant2 : Constant  Value=2*pi*fnom
  Constant4 : Constant  Value=2*pi
  Constant5 : Constant  Value=690*(1.414/1.732)
  Discrete-Time Integrator1 : DiscreteIntegrator  gainval=Ki_q  SampleTime=Ts  ICPrevOutput=DiscIntNeverNeededParam  ICPrevScaledInput=DiscIntNeverNeededParam
  Discrete-Time Integrator4 : DiscreteIntegrator  SampleTime=-1  ICPrevOutput=DiscIntNeverNeededParam  ICPrevScaledInput=DiscIntNeverNeededParam
  Discrete-Time Integrator5 : DiscreteIntegrator  SampleTime=-1  ICPrevOutput=DiscIntNeverNeededParam  ICPrevScaledInput=DiscIntNeverNeededParam
  First-Order Filter1 : spsFirstOrderFilterLib/First-Order Filter  FilterType=Lowpass  Tc=tau  Ts=Ts  Initialize=off  Vac_Init=[0, 0, 60]  Vdc_Init=0  PlotResponse=off  FreqRange="[0,  200,  1]"
  Gain10 : Gain  Gain=mp*2*pi*fnom
  Gain12 : Gain  Gain=1/(mp)
  Math Function : Math  Operator=mod  SignedPower=on
  "Power (3ph, Instantaneous)" : spsPower3phInstantaneousLib/Power (3ph, Instantaneous)
  Product : Product
  Product1 : Product
  Ramp : simulink/Sources/Ramp  slope=50  start=0  InitialOutput=0
  Saturation : Saturate  UpperLimit=563.5  LowerLimit=0  LinearizeAsGain=off  ZeroCross=off
  Saturation1 : Saturate  UpperLimit=563.5*1.1  LowerLimit=563.5*0.9  LinearizeAsGain=off  ZeroCross=off
  Scope : Scope  NumInputPorts=2
  Scope2 : Scope
  Step : Step  Time=0  SampleTime=0
  Sum1 : Sum  Inputs=|++  InputSameDT=on  SaturateOnIntegerOverflow=on
  Sum10 : Sum  Inputs=-|+||
  Sum11 : Sum  Inputs=|++
  Sum2 : Sum  Inputs=|-+  InputSameDT=on  SaturateOnIntegerOverflow=on
  Sum3 : Sum  Inputs=++|  InputSameDT=on  SaturateOnIntegerOverflow=on
  Sum4 : Sum  Inputs=|-+  InputSameDT=on  SaturateOnIntegerOverflow=on
  Sum5 : Sum  Inputs=|++  InputSameDT=on  SaturateOnIntegerOverflow=on
  T_power : powerlib_extras/Discrete  Control Blocks/Discrete 1st-Order Filter  FilterType=Lowpass  Tc=tau  Ts=Ts  Initialize=on  Vac_Init=[0 0 0]  Vdc_Init=1  PlotResponse=off  param1=[1 500 0.1]
  nq : Gain  Gain=nq
  nq1 : Gain  Gain=0
  nq2 : Gain
  nq3 : Gain  Gain=0
  Theta : Outport
  Vd_ref : Outport  Port=2
  Vq_ref : Outport  Port=3
  w_droop : Outport  Port=4
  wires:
  Constant4/1 -> Math Function/2
  T_power/1 -> Sum2/1
  Pref_pu/1 -> Sum2/2
  Vabc_pu/1 -> [Vabc_pu], "Power (3ph, Instantaneous)"/1
  Iabc_pu/1 -> "Power (3ph, Instantaneous)"/2
  "Power (3ph, Instantaneous)"/1 -> [P_meas]
  "Power (3ph, Instantaneous)"/2 -> [Q_meas]
  [P_meas] -> T_power/1
  Math Function/1 -> Theta/1
  Discrete-Time Integrator5/1 -> Product/1, Gain12/1  "θ' = ω"
  Sum2/1 -> Sum10/2
  Discrete-Time Integrator4/1 -> Math Function/1  "θ"
  Sum10/1 -> Gain10/1  "θ''"
  Gain10/1 -> Discrete-Time Integrator5/1
  Gain12/1 -> Sum10/1
  Sum11/1 -> Discrete-Time Integrator4/1, w_droop/1
  Constant2/1 -> Sum11/2
  nq/1 -> Sum3/2
  Sum4/1 -> nq/1, Discrete-Time Integrator1/1
  First-Order Filter1/1 -> Scope/2, Sum4/1
  [Q_meas] -> Scope/1, First-Order Filter1/1
  Qref_pu/1 -> Sum4/2
  Constant/1 -> Vq_ref/1
  Discrete-Time Integrator1/1 -> nq1/1
  nq1/1 -> Sum3/1
  Sum3/1 -> Product1/2
  Product1/1 -> Sum5/1
  Ramp/1 -> Saturation/1
  Sum5/1 -> Saturation1/1
  Saturation1/1 -> Scope2/1, Vd_ref/1
  Product/1 -> Sum11/1
  Step/1 -> Product/2, Product1/1
  Sum1/1 -> Sum5/2
  Constant5/1 -> nq2/1
  nq2/1 -> Sum1/2
  Saturation/1 -> nq3/1
  nq3/1 -> Sum1/1
